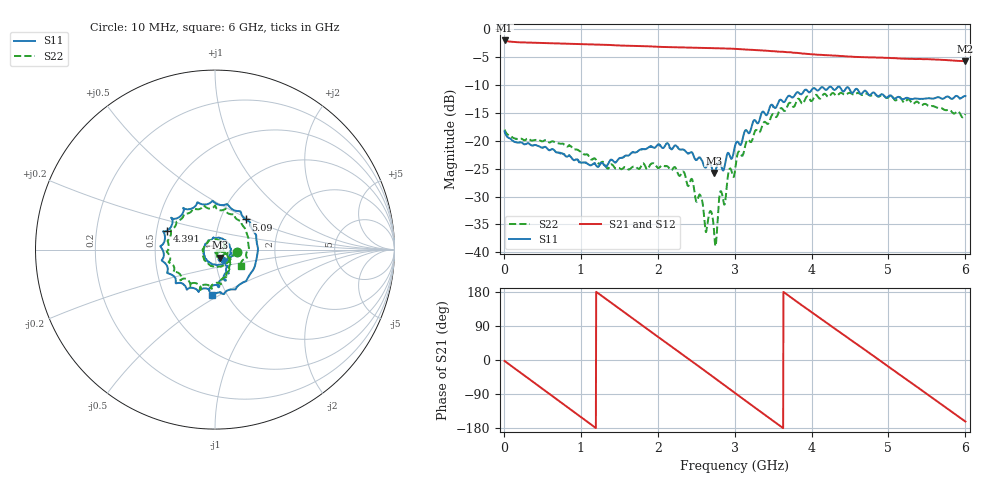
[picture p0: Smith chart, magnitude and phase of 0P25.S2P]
!Agilent Technologies,E5071C,MY46316741,A.11.02
!Date: Tue Oct 20 14:43:03 2020
!Data & Calibration Information:
!Freq	S11:SOLT4(ON)	S21:SOLT4(ON)	S12:SOLT4(ON)	S22:SOLT4(ON)
!PortZ  Port1:50+j0  Port2:50+j0
!Above PortZ is port z conversion or system Z0 setting when saving the data.
!When reading, reference impedance value at option line is always used.
# Hz S dB R 50
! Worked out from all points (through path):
!   1561 points, 10 MHz to 6 GHz, reference 50 ohm
!   highest |S21| = -2.01 dB at 10 MHz (marker M1); lowest = -5.7 dB at 6 GHz (marker M2)
!   group delay of S21, straight-line fit = 408 ps
!   lowest |S11| = -25.8 dB at 2.729 GHz (marker M3), VSWR 1.11, Z = 52.5 - j4.65 ohm
!   |S11| at or under -10 dB: start of sweep to end of sweep
!   |S22| runs from -38.9 to -11.4 dB; largest |S21 - S12| = 0.0058
!   S11 on the Smith chart (normalised r, x): 10 MHz: 1.27, -0.04; 4.391 GHz: 0.57, +0.13; 5.09 GHz: 1.32, +0.47; 6 GHz: 0.85, -0.46
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1e7  -18.33 -7.4  -2.01 -2.4  -2.06 -2.4  -17.99 -6.7
2.557436e8  -20.55 -40.3  -2.37 -39.3  -2.41 -39.2  -19.86 -33.0
5.322051e8  -21.09 -81.8  -2.47 -80.5  -2.51 -80.5  -19.89 -68.6
7.5875e8  -22.28 -119.9  -2.56 -114.3  -2.58 -114.3  -20.50 -101.9
1.012173e9  -23.95 -171.4  -2.65 -152.1  -2.68 -152.1  -22.14 -144.7
1.288635e9  -24.09 125.5  -2.77 166.8  -2.78 166.8  -23.75 156.1
1.584295e9  -22.64 56.6  -2.95 123.1  -2.97 123.0  -24.75 82.3
2.006667e9  -20.61 -12.9  -3.15 60.7  -3.16 60.7  -24.90 -7.7
2.371442e9  -22.03 -54.4  -3.29 7.2  -3.31 6.9  -27.10 -58.3
2.728538e9  -25.79 -59.3  -3.39 -45.7  -3.43 -45.9  -35.51 -11.5
2.759256e9  -24.95 -65.5  -3.41 -50.2  -3.43 -50.5  -38.31 -34.6
2.816853e9  -24.13 -46.6  -3.43 -58.8  -3.47 -59.1  -29.04 -9.4
3.005e9  -20.94 -51.0  -3.52 -87.0  -3.56 -87.2  -25.38 -18.5
3.239224e9  -16.62 -62.2  -3.71 -121.9  -3.74 -122.0  -19.37 -40.3
3.527205e9  -14.12 -88.6  -3.96 -164.6  -3.98 -164.7  -15.66 -68.6
4.007173e9  -10.77 -152.4  -4.49 125.3  -4.50 125.2  -12.83 -134.3
4.391147e9  -10.86 158.3  -4.80 70.0  -4.83 69.8  -11.43 -177.9
4.713686e9  -11.19 109.3  -5.02 23.9  -5.05 23.7  -11.56 143.5
5.001667e9  -12.02 59.0  -5.13 -17.9  -5.16 -17.9  -12.16 106.5
5.089981e9  -12.41 44.6  -5.19 -30.7  -5.23 -30.6  -12.77 96.8
5.523872e9  -12.36 -27.0  -5.37 -93.3  -5.39 -93.3  -13.77 42.6
6e9  -11.99 -94.3  -5.74 -162.4  -5.73 -162.4  -15.22 -31.9
